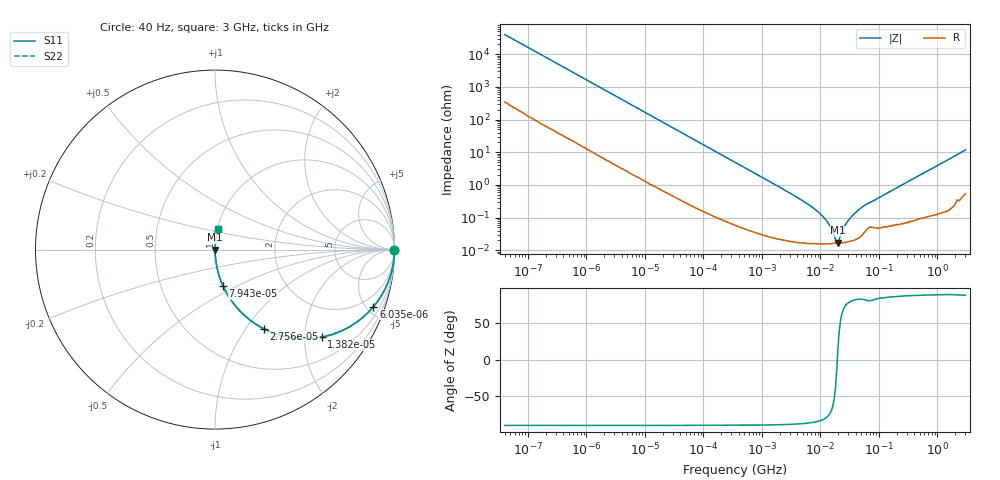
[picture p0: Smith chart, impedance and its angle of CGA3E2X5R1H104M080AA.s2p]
! S-parameter Generated by TDK Corporation
! Copyright(C) 2015 TDK Corporation.
! All Rights Reserved.
! TDK P/N: CGA3E2X5R1H104M080AA (Multilayer Ceramic Chip Capacitors)
! Property: C=100nF
! Size(LxWxT): 1.6x0.8x0.8mm, 0.063x0.031x0.031inches
! Model Type: s2p (Touchstone File Format Version 1.0)
! Frequency: DC=Yes Start=0.00004MHz Stop=3000MHz 396points Log-sweep
! Note: This model was converted from impedance.
! Model Generated on Jun. 23, 2015
! Hash(MD5):
! Port Assignments:
!  1 ---| |--- 2
! Applicable Conditions:
!  Temperature = 25 degC
!  DC Bias Voltage = 0 V
!  Small Signal Operation
! Terms and conditions regarding TDK Simulation Models
! (1)This simulation model is being provided solely for informational purposes. Please refer to the specifications of the products in terms of detailed characteristics of such products.
! (2)In no event shall TDK Corporation of any of its subsidiaries be liable for any loss or damage arising, directly or indirectly,
!  From any information contained in this simulation model, including, but not limited to loss or damages arising from any inaccuracies, omissions or errors in connection with such information.
! (3)Any and all copyrights on this simulation model are owned by TDK Corporation.
!  Duplication or redistribution of this simulation model without prior written permission from TDK Corporation is prohibited.
! (4)This simulation model is subject to any modification or change without any prior notice.
! (5)Neither TDK Corporation nor any of its subsidiaries shall make any warranty, express or implied,
!  Including but not limited to the correctness, implied warranties of merchantability and fitness for a particular purpose with respect to this simulation models.
! (6)The use of this simulation model shall be deemed to have consented to the terms and conditions hereof.
# MHz S MA R 50
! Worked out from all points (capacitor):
!   395 points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, 40 Hz to 3 GHz, reference 50 ohm
!   read as one part in series: C = 98.1 nF near 41.88 Hz
!   lowest |Z| = 16.9 mohm at 19.88 MHz (marker M1)
!   series resonance near 19.43 MHz, so ESL is about 680 pH
!   S11 on the Smith chart (normalised r, x): 40 Hz: open; 6.035 kHz: 1.04, -5.53; 13.82 kHz: 1.02, -2.43; 27.56 kHz: 1.01, -1.22; 79.43 kHz: 1.00, -0.43; 3 GHz: 1.01, +0.24
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4e-05  1 -0.1  0.00247 89.4  0.00247 89.4  1 -0.1
0.000834128  0.9983 -2.9  0.05036 86.7  0.05036 86.7  0.9983 -2.9
0.002404055  0.9886 -8.2  0.1429 81.3  0.1429 81.3  0.9886 -8.2
0.006035228  0.9382 -19.8  0.339 69.7  0.339 69.7  0.9382 -19.8
0.01381873  0.7688 -39.3  0.6335 50.2  0.6335 50.2  0.7688 -39.3
0.01739424  0.6917 -45.8  0.7168 43.8  0.7168 43.8  0.6917 -45.8
0.02756005  0.5192 -58.3  0.8505 31.3  0.8505 31.3  0.5192 -58.3
0.04572378  0.3452 -69.3  0.9357 20.2  0.9357 20.2  0.3452 -69.3
0.07943131  0.2081 -77.5  0.9763 12.0  0.9763 12.0  0.2081 -77.5
0.3464102  0.04927 -86.5  0.9982 2.8  0.9982 2.8  0.04927 -86.5
2.877491  0.005897 -87.8  0.9998 0.3  0.9998 0.3  0.005897 -87.8
7.22376  0.002082 -85.5  0.9998 0.1  0.9998 0.1  0.002082 -85.5
12.54911  0.0008253 -78.9  0.9998 0.0  0.9998 0.0  0.0008253 -78.9
15.08561  0.0004858 -71.0  0.9998 0.0  0.9998 0.0  0.0004858 -71.0
18.98891  0.0001702 -14.2  0.9998 0.0  0.9998 0.0  0.0001702 -14.2
19.88326  0.0001686 14.4  0.9998 -0.0  0.9998 -0.0  0.0001686 14.4
26.2067  0.0005686 72.2  0.9998 -0.0  0.9998 -0.0  0.0005686 72.2
36.16801  0.001205 80.6  0.9998 -0.1  0.9998 -0.1  0.001205 80.6
57.30589  0.002388 81.1  0.9996 -0.1  0.9996 -0.1  0.002388 81.1
150.6385  0.00613 84.6  0.9994 -0.3  0.9994 -0.3  0.00613 84.6
994.0817  0.03886 85.9  0.998 -2.2  0.998 -2.2  0.03886 85.9
3000  0.1167 80.7  0.9879 -6.7  0.9879 -6.7  0.1167 80.7
